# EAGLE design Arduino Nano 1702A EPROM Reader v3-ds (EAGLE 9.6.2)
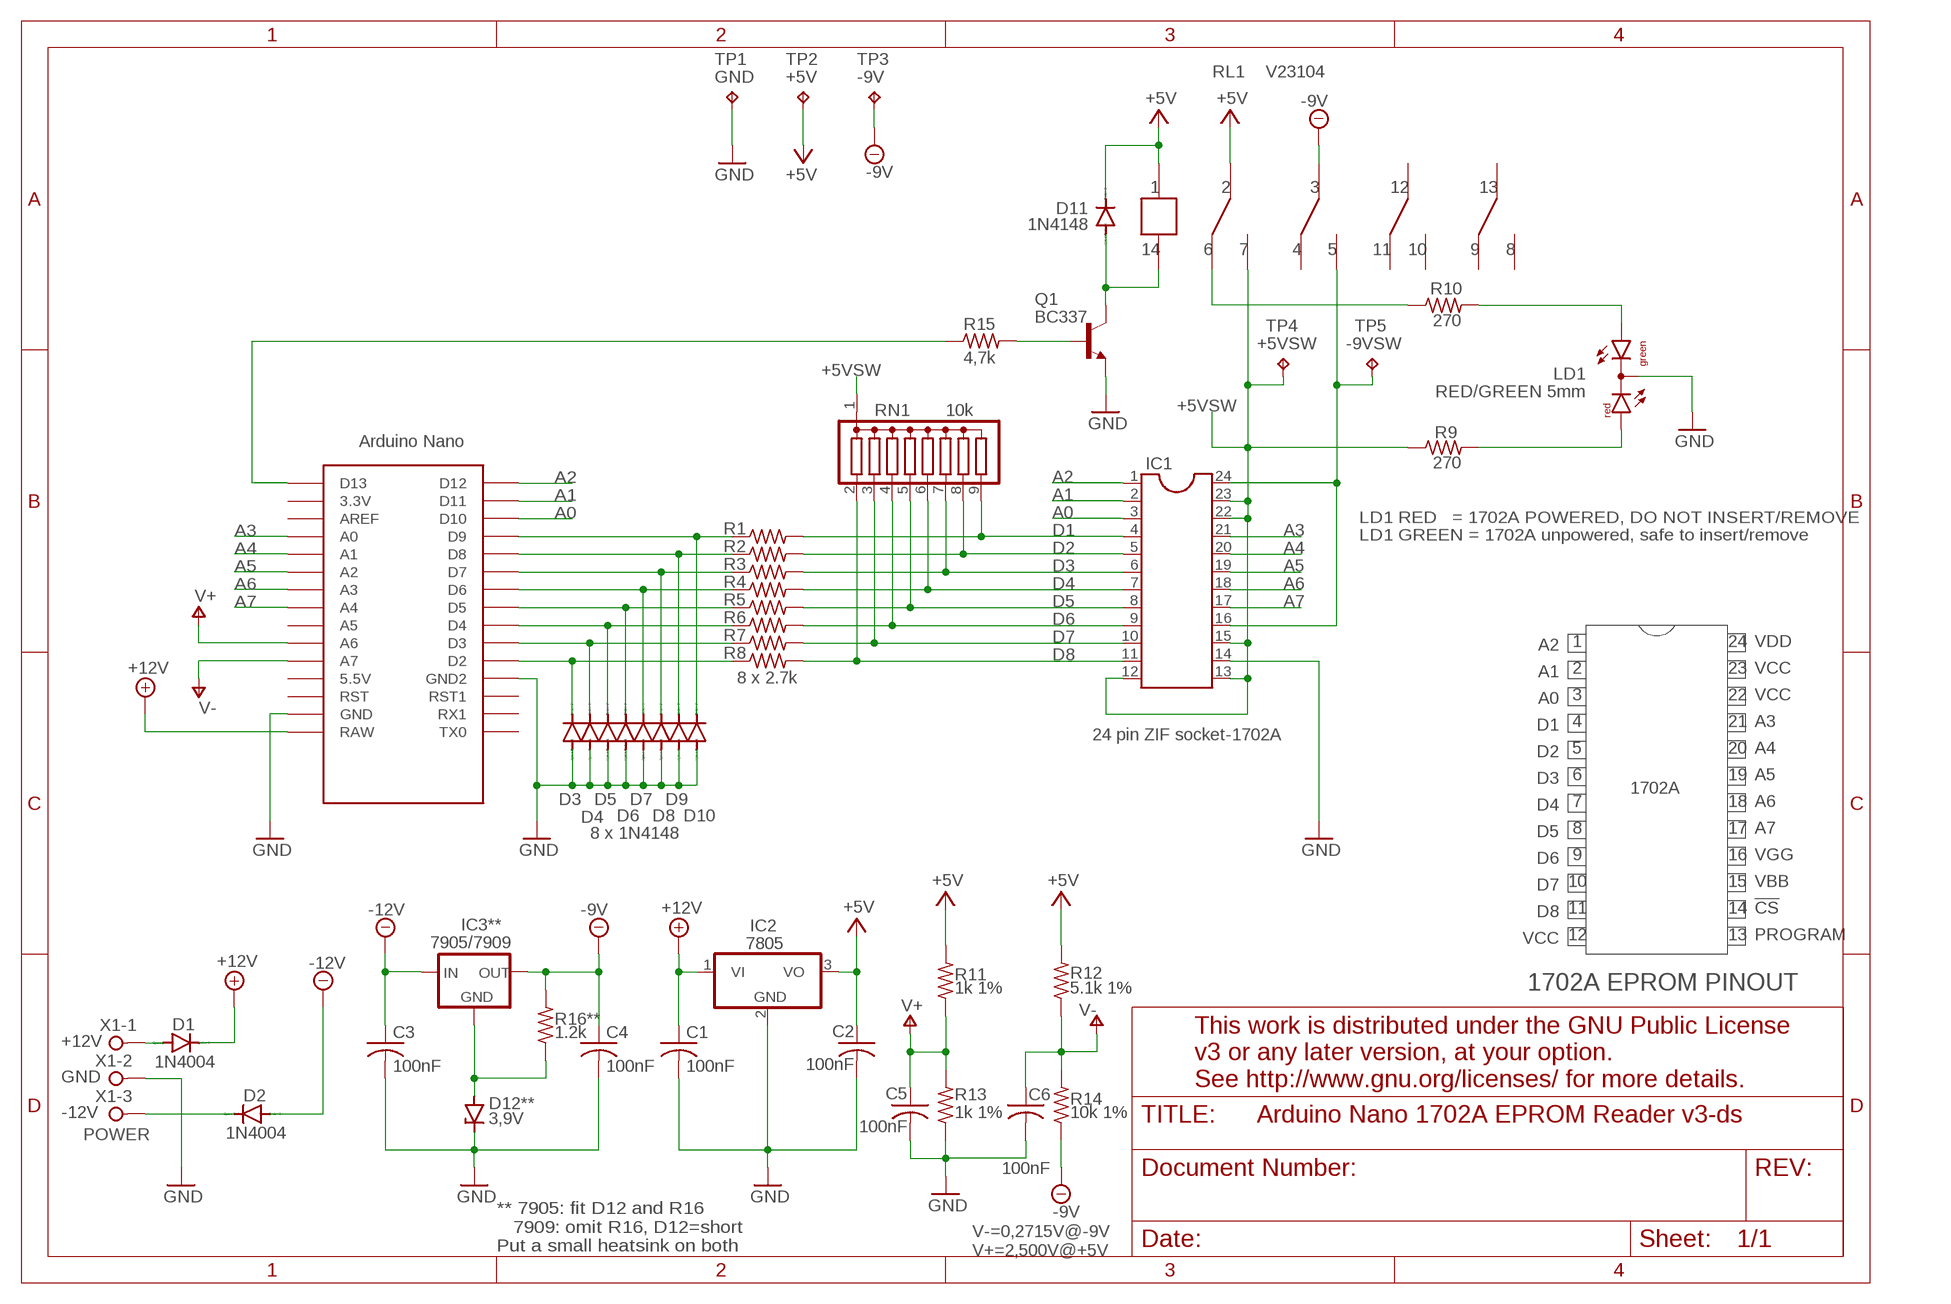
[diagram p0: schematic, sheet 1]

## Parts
C1  100nF  RCL_C-US050-025X075  [RCL_C050-025X075]
C2  100nF  RCL_C-US050-025X075  [RCL_C050-025X075]
C3  100nF  RCL_C-US050-025X075  [RCL_C050-025X075]
C4  100nF  RCL_C-US050-025X075  [RCL_C050-025X075]
C5  100nF  RCL_C-US050-025X075  [RCL_C050-025X075]
C6  100nF  RCL_C-US050-025X075  [RCL_C050-025X075]
D1  1N4004  ARDUINO-NANO-1702A-EPROM-READER-V2_1N4004  [ARDUINO-NANO-1702A-EPROM-READER-V2_DO41-10]
D2  1N4004  ARDUINO-NANO-1702A-EPROM-READER-V2_1N4004  [ARDUINO-NANO-1702A-EPROM-READER-V2_DO41-10]
D3  8 x 1N4148  DIODE_1N4148DO35-10  [DIODE_DO35-10]
D4  DIODE_1N4148DO35-10  [DIODE_DO35-10]
D5  DIODE_1N4148DO35-10  [DIODE_DO35-10]
D6  DIODE_1N4148DO35-10  [DIODE_DO35-10]
D7  DIODE_1N4148DO35-10  [DIODE_DO35-10]
D8  DIODE_1N4148DO35-10  [DIODE_DO35-10]
D9  DIODE_1N4148DO35-10  [DIODE_DO35-10]
D10  1N4148  DIODE_1N4148DO35-10  [DIODE_DO35-10]
D11  1N4148  DIODE_1N4148DO35-10  [DIODE_DO35-10]
D12**  3,9V  DIODE_ZPD  [DIODE_DO35Z10]
IC1  24 pin ZIF socket-1702A  IC-PACKAGE_DIL24-6  [IC-PACKAGE_DIL24-6]
IC2  7805  LINEAR_7805TV  [LINEAR_TO220V]
IC3**  7905/7909  V-REG_79XXS  [V-REG_79XXS]
LD1  RED/GREEN 5mm  LED_DUOLED-RG-C  [LED_DUOLED-C-5MM]
Q1  BC337  TRANSISTOR-NPN_BC237  [TRANSISTOR-NPN_TO92]
R1  RCL_R-US_0207/10  [RCL_0207/10]
R2  RCL_R-US_0207/10  [RCL_0207/10]
R3  RCL_R-US_0207/10  [RCL_0207/10]
R4  RCL_R-US_0207/10  [RCL_0207/10]
R5  RCL_R-US_0207/10  [RCL_0207/10]
R6  RCL_R-US_0207/10  [RCL_0207/10]
R7  RCL_R-US_0207/10  [RCL_0207/10]
R8  8 x 2.7k  RCL_R-US_0207/10  [RCL_0207/10]
R9  270  RCL_R-US_0207/10  [RCL_0207/10]
R10  270  RCL_R-US_0207/10  [RCL_0207/10]
R11  1k 1%  RCL_R-US_0207/10  [RCL_0207/10]
R12  5.1k 1%  RCL_R-US_0207/10  [RCL_0207/10]
R13  1k 1%  RCL_R-US_0207/10  [RCL_0207/10]
R14  10k 1%  RCL_R-US_0207/10  [RCL_0207/10]
R15  4,7k  RCL_R-US_0207/10  [RCL_0207/10]
R16**  1.2k  RCL_R-US_0207/10  [RCL_0207/10]
RL1  V23104  ARDUINO-NANO-1702A-EPROM-READER-V2_V23104  [ARDUINO-NANO-1702A-EPROM-READER-V2_V23104]
RN1  10k  G08R  [SIL9]
TP1  TPPAD1-13Y  [P1-13Y]
TP2  TPPAD1-13Y  [P1-13Y]
TP3  TPPAD1-13Y  [P1-13Y]
TP4  +5VSW  TPPAD1-13Y  [P1-13Y]
TP5  TPPAD1-13Y  [P1-13Y]
U$1  ARDUINO-CLONE_NANO  [ARDUINO-CLONE_NANO]
X1  POWER  CON-WAGO-508_W237-3E  [CON-WAGO-508_W237-3E]

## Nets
+5V: C2.1 D11.C IC2.3(VO) R11.2 R12.2 RL1.P$1 RL1.P$2 TP2.TP
+5VSW: IC1.12 IC1.13 IC1.15 IC1.22 IC1.23 R9.1 RL1.P$7 RN1.1 TP4.TP
+12V: C1.1 D1.C IC2.1(VI) U$1.RAW
-9V: C4.1 IC3**.OUT R14.1 R16**.2 RL1.P$3 TP3.TP
-9VSW: IC1.16 IC1.24 RL1.P$5 TP5.TP
-12V: C3.1 D2.A IC3**.IN
A0: IC1.3 U$1.D10
A1: IC1.2 U$1.D11
A2: IC1.1 U$1.D12
A3: IC1.21 U$1.A0
A4: IC1.20 U$1.A1
A5: IC1.19 U$1.A2
A6: IC1.18 U$1.A3
A7: IC1.17 U$1.A4
D1: IC1.4 R1.2 RN1.9
D2: IC1.5 R2.2 RN1.8
D3: IC1.6 R3.2 RN1.7
D4: IC1.7 R4.2 RN1.6
D5: IC1.8 R5.2 RN1.5
D6: IC1.9 R6.2 RN1.4
D7: IC1.10 R7.2 RN1.3
D8: IC1.11 R8.2 RN1.2
GND: C1.2 C2.2 C3.2 C4.2 C5.2 C6.2 D3.A D4.A D5.A D6.A D7.A D8.A D9.A D10.A D12**.C IC1.14 IC2.2(GND) LD1.C Q1.1(E) R13.1 TP1.TP U$1.GND U$1.GND1(GND2) X1.2
N$1: D1.A X1.1
N$2: D2.C X1.3
N$3: D12**.A IC3**.GND R16**.1
N$4: D11.A Q1.3(C) RL1.P$14
N$5: LD1.AR R9.2
N$6: D3.C R8.1 U$1.D2
N$7: D4.C R7.1 U$1.D3
N$8: D5.C R6.1 U$1.D4
N$9: D6.C R5.1 U$1.D5
N$10: D7.C R4.1 U$1.D6
N$11: D8.C R3.1 U$1.D7
N$12: D9.C R2.1 U$1.D8
N$13: D10.C R1.1 U$1.D9
N$15: LD1.AX(AG) R10.2
N$16: R10.1 RL1.P$6
N$17: Q1.2(B) R15.2
N$18: R15.1 U$1.D13
V+: C5.1 R11.1 R13.2 U$1.A6
V-: C6.1 R12.1 R14.2 U$1.A7
Unconnected: RL1.P$4 RL1.P$8 RL1.P$9 RL1.P$10 RL1.P$11 RL1.P$12 RL1.P$13 U$1.3.3V U$1.5V(5.5V) U$1.A5 U$1.AREF U$1.RST U$1.RST1 U$1.RX1 U$1.TX0

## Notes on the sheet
- LD1 RED   = 1702A POWERED, DO NOT INSERT/REMOVE
  LD1 GREEN = 1702A unpowered, safe to insert/remove
- A2
- 1 | 24 | VDD
- A1
- 2 | 23 | VCC
- A0
- 3 | 22 | VCC
- D1
- 4 | 21 | A3
- D2
- 5 | 20 | A4
- D3
- 6 | 19 | A5
- D4 | 1702A
- 7 | 18 | A6
- D5
- 8 | 17 | A7
- D6
- 9 | 16 | VGG
- D7
- 10 | 15 | VBB
- D8
- 11 | 14 | !CS!
- VCC
- 12 | 13 | PROGRAM
- 1702A EPROM PINOUT
- +12V
- GND
- This work is distributed under the GNU Public License
  v3 or any later version, at your option.
  See http://www.gnu.org/licenses/ for more details.
- -12V
- ** 7905: fit D12 and R16
     7909: omit R16, D12=short
  Put a small heatsink on both
- V-=0,2715V@-9V
  V+=2,500V@+5V

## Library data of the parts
C1-C6 = Arduino Nano 1702A EPROM Reader v3:RCL_C-US: CAPACITOR, American symbol; SPICEPREFIX: C
D1 D2 = Arduino Nano 1702A EPROM Reader v3:ARDUINO-NANO-1702A-EPROM-READER-V2_1N4004: DIODE
D3-D11 = Arduino Nano 1702A EPROM Reader v3:DIODE_1N4148: DIODE
D12** = Arduino Nano 1702A EPROM Reader v3:DIODE_ZPD: Z DIODE
IC1 = Arduino Nano 1702A EPROM Reader v3:IC-PACKAGE_DIL24: Dual In Line
IC2 = Arduino Nano 1702A EPROM Reader v3:LINEAR_78*: Positive VOLTAGE REGULATOR Source: http://cache.national.com/ds/LM/LM78L05.pdf http://www.fairchildsemi.com/ds/LM/LM7805.pdf
IC3** = Arduino Nano 1702A EPROM Reader v3:V-REG_79XXS: VOLTAGE REGULATOR
LD1 = Arduino Nano 1702A EPROM Reader v3:LED_DUOLED-RG-C: DUO LED 2 colors (red/green), 5 mm, round, common Cathode www.ligitek.com or other producers.
Q1 = Arduino Nano 1702A EPROM Reader v3:TRANSISTOR-NPN_BC237: NPN Transistor
R1-R15 R16** = Arduino Nano 1702A EPROM Reader v3:RCL_R-US_: RESISTOR, American symbol; SPICEPREFIX: R
RL1 = Arduino Nano 1702A EPROM Reader v3:ARDUINO-NANO-1702A-EPROM-READER-V2_V23104
RN1 = resistor-sil:G08R: SIL RESISTOR; OC_FARNELL: unknown; OC_NEWARK: unknown
TP1 = testpad:TP: Test pad; TP_SIGNAL_NAME: GND
TP2 = testpad:TP: Test pad; TP_SIGNAL_NAME: +5V
TP3 = testpad:TP: Test pad; TP_SIGNAL_NAME: -9V
TP4 = testpad:TP: Test pad; TP_SIGNAL_NAME: +5VSW
TP5 = testpad:TP: Test pad; TP_SIGNAL_NAME: -9VSW
U$1 = Arduino Nano 1702A EPROM Reader v3:ARDUINO-CLONE_NANO: Arduino Nano
X1 = Arduino Nano 1702A EPROM Reader v3:CON-WAGO-508_W237-3E: WAGO SREW CLAMP; OC_FARNELL: unknown; OC_NEWARK: unknown

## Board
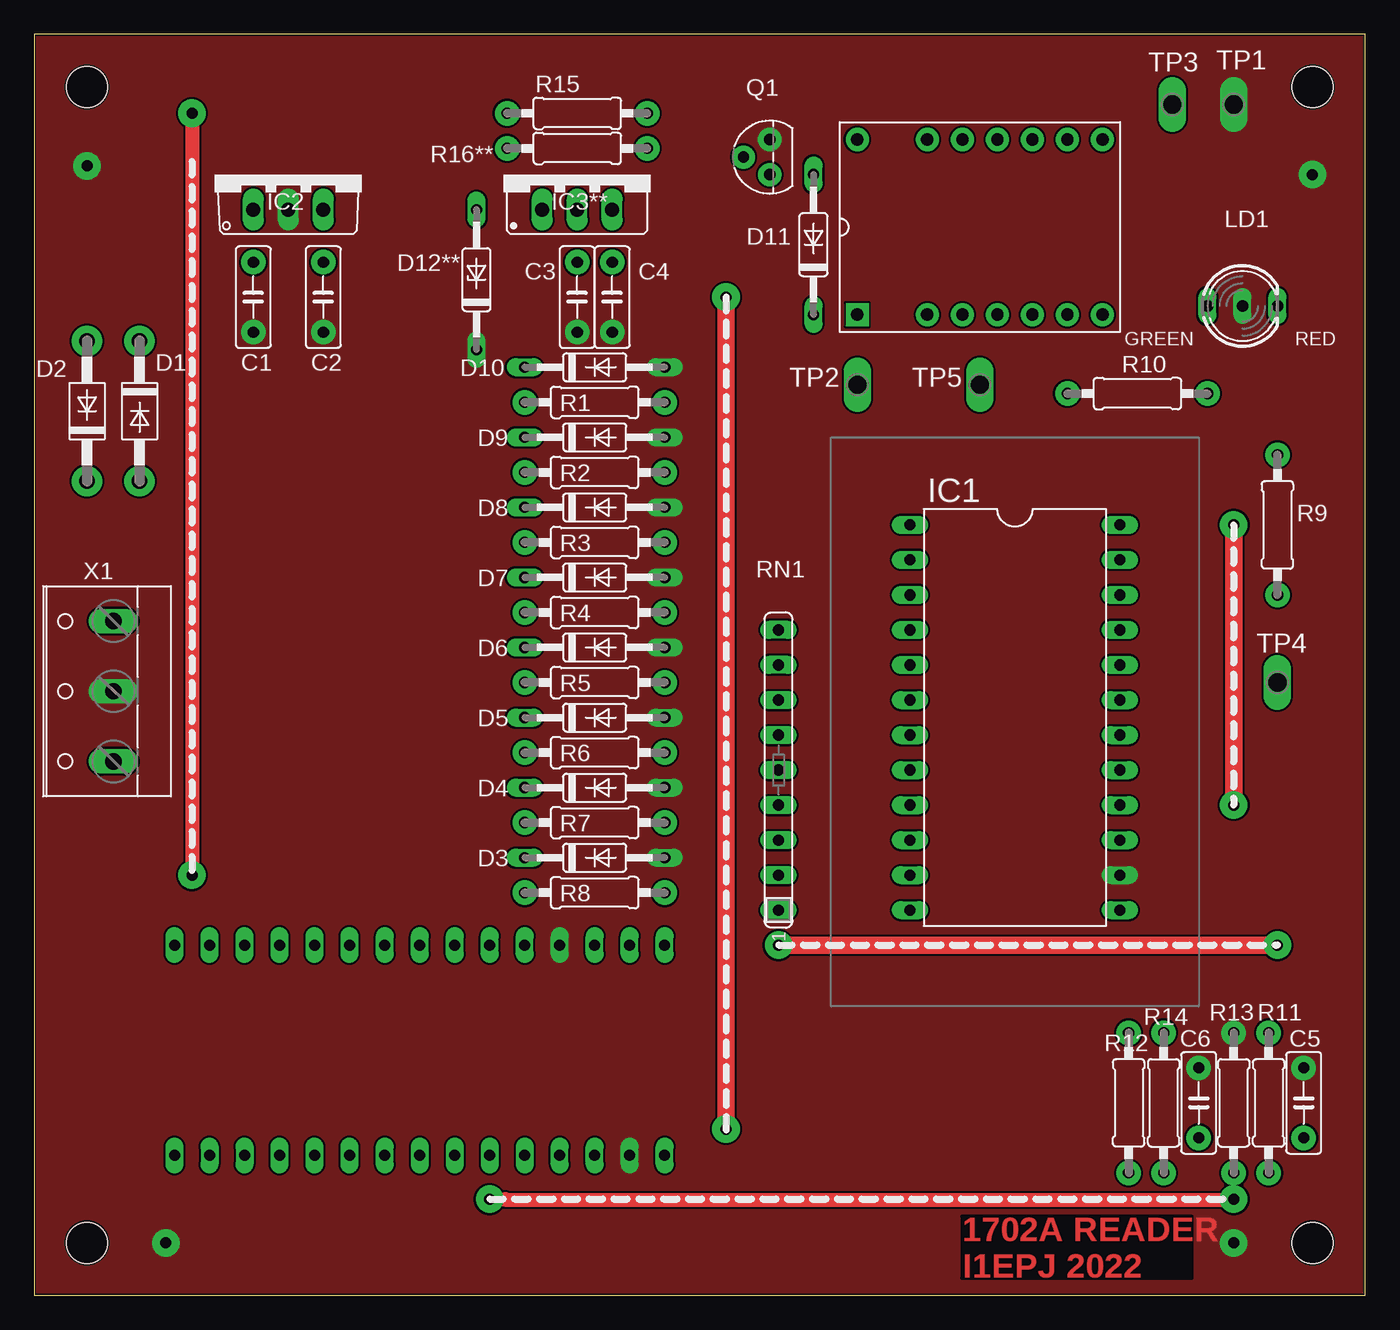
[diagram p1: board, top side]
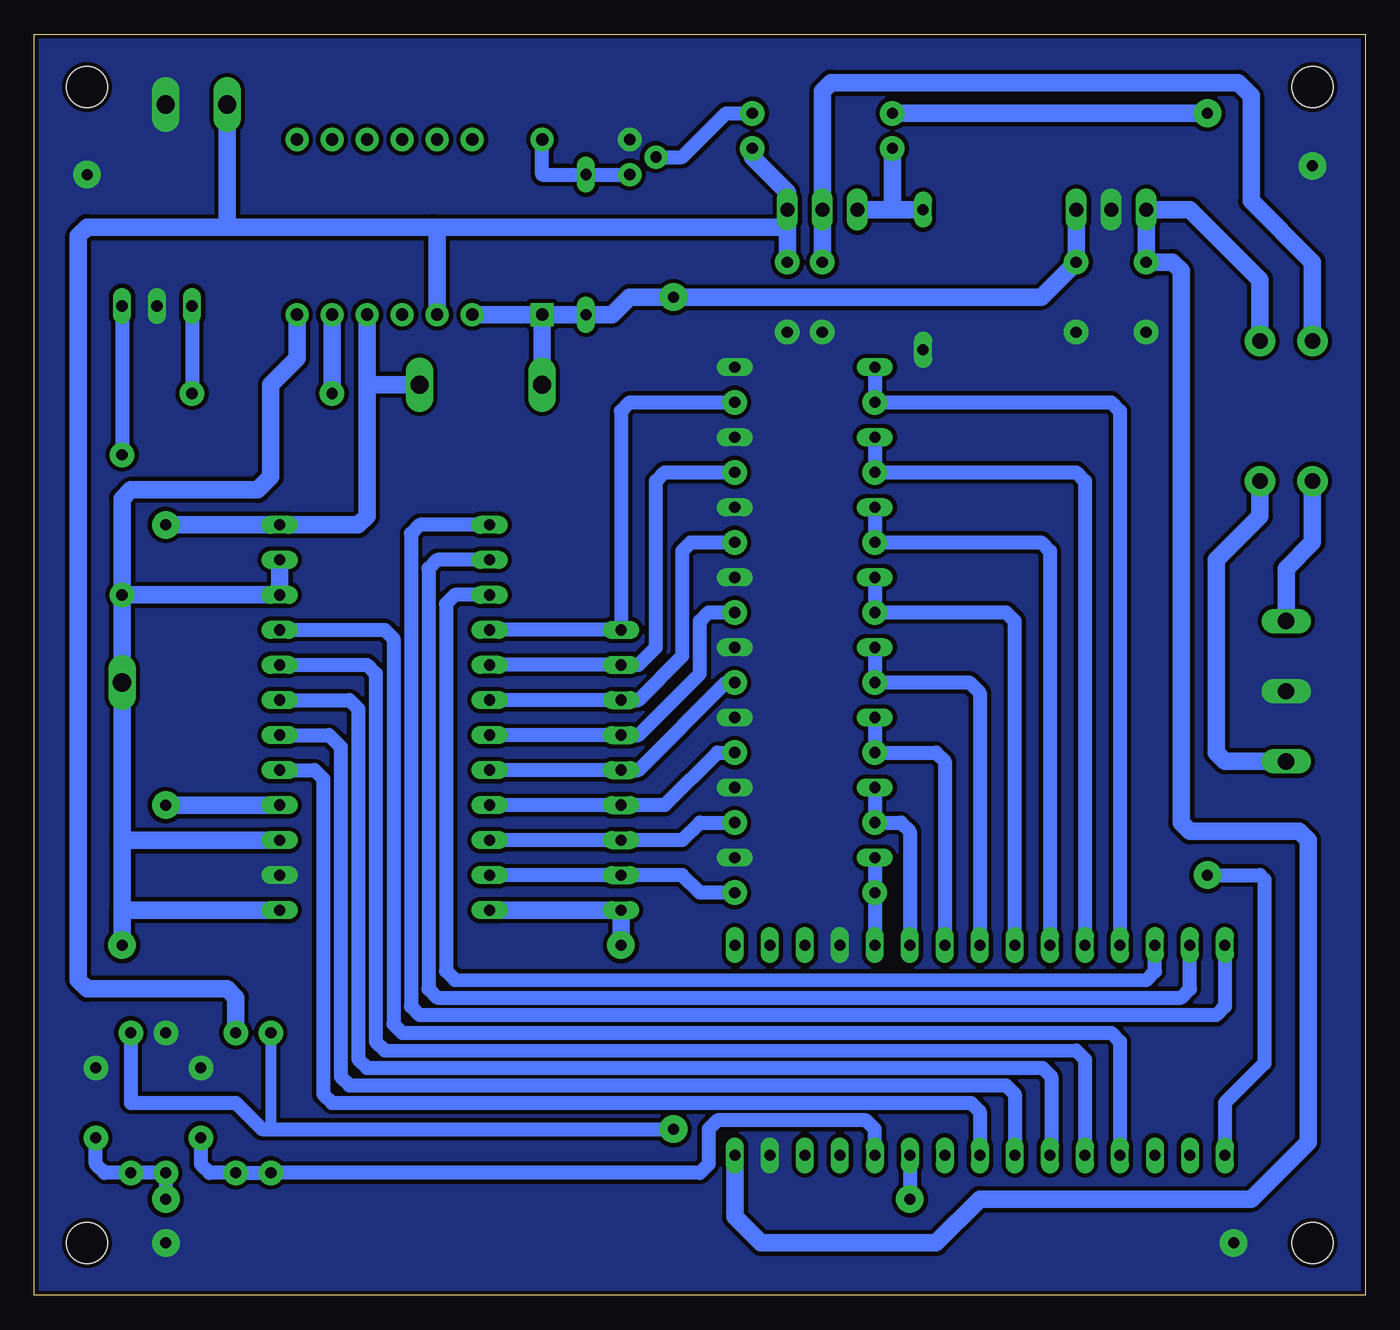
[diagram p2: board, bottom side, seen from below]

Size 96.52 x 91.44 mm. Coordinates in mm from the lower left corner, seen from the top.
Outline: 0,0 96.52,0 96.52,91.44 0,91.44 0,0
Copper layers (1*16): Top 0.035mm / dielectric 1.5mm / Bottom 0.035mm
Design rules "default *": minimum track width 6mil, minimum drill 0.35mm, track to track 6mil, track to pad 6mil, pad to pad 6mil, via to via 6mil, smd to smd 6mil, copper to edge 5mil, drill to drill 6mil, minimum pad ring 10mil, minimum via ring 8mil, stop-mask expansion 4mil, vias tented up to drill 0mil, thermal gap 0mil
Holes 3 mm at 92.71,3.81 3.81,3.81 3.81,87.63 92.71,87.63

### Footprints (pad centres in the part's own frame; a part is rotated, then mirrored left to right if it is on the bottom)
RCL_C050-025X075 = drill 0.813 pad 1.778: 1 -2.54,0; 2 2.54,0
ARDUINO-NANO-1702A-EPROM-READER-V2_DO41-10 = drill 1.118 pad 2.184: A 5.08,0; C -5.08,0
DIODE_DO35-10 = drill 0.813 long: A 5.08,0; C -5.08,0
DIODE_DO35Z10 = drill 0.813 long: A 5.08,0; C -5.08,0
IC-PACKAGE_DIL24-6 = drill 0.813 long: 1 -13.97,-7.62; 2 -11.43,-7.62; 3 -8.89,-7.62; 4 -6.35,-7.62; 5 -3.81,-7.62; 6 -1.27,-7.62; 7 1.27,-7.62; 8 3.81,-7.62; 9 6.35,-7.62; 10 8.89,-7.62; 11 11.43,-7.62; 12 13.97,-7.62; 13 13.97,7.62; 14 11.43,7.62; 15 8.89,7.62; 16 6.35,7.62; 17 3.81,7.62; 18 1.27,7.62; 19 -1.27,7.62; 20 -3.81,7.62; 21 -6.35,7.62; 22 -8.89,7.62; 23 -11.43,7.62; 24 -13.97,7.62
LINEAR_TO220V = drill 1.016 long: 1 -2.54,-2.54; 2 0,-2.54; 3 2.54,-2.54
V-REG_79XXS = drill 1.016 long: GND -2.54,-2.54; IN 0,-2.54; OUT 2.54,-2.54
LED_DUOLED-C-5MM = drill 0.813 long: AR 2.54,0; AX -2.54,0; C 0,0
TRANSISTOR-NPN_TO92 = drill 0.813 pad 1.676: 1 1.27,0; 2 0,1.905; 3 -1.27,0
RCL_0207/10 = drill 0.813 pad 1.778: 1 -5.08,0; 2 5.08,0
ARDUINO-NANO-1702A-EPROM-READER-V2_V23104 = drill 0.9 pad 1.676 square: P$1 -10.16,0 | drill 0.9 pad 1.676: P$2 -5.08,0; P$3 -2.54,0; P$4 0,0; P$5 2.54,0; P$6 5.08,0; P$7 7.62,0; P$8 7.62,12.7; P$9 5.08,12.7; P$10 2.54,12.7; P$11 0,12.7; P$12 -2.54,12.7; P$13 -5.08,12.7; P$14 -10.16,12.7
SIL9 = drill 0.813 long: 1 -10.16,0; 2 -7.62,0; 3 -5.08,0; 4 -2.54,0; 5 0,0; 6 2.54,0; 7 5.08,0; 8 7.62,0; 9 10.16,0
P1-13Y = drill 1.321 pad 1.905 long: TP 0,0
ARDUINO-CLONE_NANO = drill 0.8 long: 3.3V -10.16,24.13; 5V -10.16,-1.27; A0 -10.16,19.05; A1 -10.16,16.51; A2 -10.16,13.97; A3 -10.16,11.43; A4 -10.16,8.89; A5 -10.16,6.35; A6 -10.16,3.81; A7 -10.16,1.27; AREF -10.16,21.59; D2 5.08,1.27; D3 5.08,3.81; D4 5.08,6.35; D5 5.08,8.89; D6 5.08,11.43; D7 5.08,13.97; D8 5.08,16.51; D9 5.08,19.05; D10 5.08,21.59; D11 5.08,24.13; D12 5.08,26.67; D13 -10.16,26.67; GND -10.16,-6.35; GND1 5.08,-1.27; RAW -10.16,-8.89; RST -10.16,-3.81; RST1 5.08,-3.81; RX1 5.08,-6.35; TX0 5.08,-8.89
CON-WAGO-508_W237-3E = drill 1.194 long: 1 -5.08,-0.635; 2 0,-0.635; 3 5.08,-0.635

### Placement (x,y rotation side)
C1  15.88,72.39 270 top
C2  20.95,72.39 270 top
C3  39.37,72.39 270 top
C4  41.91,72.39 270 top
C5  92.08,13.97 90 top
C6  84.45,13.97 90 top
D1  7.62,64.14 270 top
D2  3.81,64.14 90 top
D3  40.64,31.75 0 top
D4  40.64,36.83 0 top
D5  40.64,41.91 0 top
D6  40.64,46.99 0 top
D7  40.64,52.07 0 top
D8  40.64,57.15 0 top
D9  40.64,62.23 0 top
D10  40.64,67.31 0 top
D11  56.52,76.2 90 top
D12**  32.07,73.66 90 top
IC1  71.12,41.91 270 top
IC2  18.41,81.28 0 top
IC3**  39.37,81.28 0 top
LD1  87.63,71.75 0 top
Q1  53.34,82.55 90 top
R1  40.64,64.77 0 top
R2  40.64,59.69 0 top
R3  40.64,54.61 0 top
R4  40.64,49.53 0 top
R5  40.64,44.45 0 top
R6  40.64,39.37 0 top
R7  40.64,34.29 0 top
R8  40.64,29.21 0 top
R9  90.17,55.88 90 top
R10  80.01,65.41 0 top
R11  89.53,13.97 90 top
R12  79.38,13.97 90 top
R13  87,13.97 270 top
R14  81.92,13.97 270 top
R15  39.37,85.72 0 top
R16**  39.37,83.19 0 top
RL1  69.85,71.12 0 top
RN1  53.98,38.1 90 top
TP1  87,86.36 0 top
TP2  59.69,66.04 0 top
TP3  82.55,86.36 0 top
TP4  90.17,44.45 180 top
TP5  68.58,66.04 0 top
U$1  36.83,20.32 90 top
X1  5.08,43.81 90 top

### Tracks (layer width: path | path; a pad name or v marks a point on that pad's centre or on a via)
+5V  (via drill 0.8 pad 2)
  Top 1.27: v50.16,72.39 v50.16,12.06
  Bottom 0.813: R12.2 79.38,12.06
  Bottom 1.016: R11.2 89.53,13.97 81.92,13.97 80.01,12.06 79.38,12.06 v50.16,12.06
  Bottom 1.27: IC2.3 C2.1 23.5,72.39 v50.16,72.39 53.34,72.39 54.61,71.12 D11.C RL1.P$1 | RL1.P$1 RL1.P$2 | TP2.TP RL1.P$1
+5VSW  (via drill 0.8 pad 2)
  Top 1.27: v90.17,25.4 v53.98,25.4
  Bottom 1.27: IC1.23 IC1.22 R9.1 | 90.17,33.02 90.17,27.94 | 90.17,33.02 IC1.15 | RL1.P$7 77.47,67.94 79.38,66.04 79.38,59.37 80.33,58.42 89.53,58.42 90.17,57.78 R9.1 | v53.98,25.4 RN1.1 IC1.12 | v90.17,25.4 90.17,27.94 | IC1.13 90.17,27.94 | R9.1 TP4.TP 90.17,33.02
+12V
  Bottom 1.27: U$1.RAW 45.72,5.71 43.81,3.81 31.11,3.81 27.94,6.99 8.26,6.99 4.13,11.11 4.13,33.02 4.76,33.66 12.7,33.66 13.34,34.29 13.34,74.3 13.97,74.93 C1.1 IC2.1 12.7,78.74 7.62,73.66 D1.C
-9V
  Bottom 1.27: 82.55,77.47 67.63,77.47 | 67.63,77.47 41.91,77.47 C4.1 IC3**.OUT 41.91,80.01 44.45,82.55 R16**.2 | 82.55,77.47 92.71,77.47 93.34,76.83 93.34,22.86 92.71,22.23 82.55,22.23 81.92,21.59 R14.1 | RL1.P$3 67.31,77.15 67.63,77.47 | TP3.TP 82.55,77.47
-9VSW  (via drill 0.8 pad 2)
  Top 1.27: v87,55.88 v87,35.56
  Bottom 1.27: 72.39,66.04 72.39,56.52 73.03,55.88 IC1.24 v87,55.88 | 72.39,66.04 RL1.P$5 | v87,35.56 IC1.16 | TP5.TP 72.39,66.04
-12V
  Bottom 1.27: C3.1 IC3**.IN 39.37,87.31 38.73,87.95 9.21,87.95 8.26,87 8.26,79.38 3.81,74.93 D2.A
A0
  Bottom 1.016: IC1.3 66.03,50.8 66.67,50.15 66.67,23.54 66.02,22.88 15.88,22.86 15.24,23.5 U$1.D10
A1
  Bottom 1.016: IC1.2 67.31,53.34 67.94,52.7 67.94,22.23 67.31,21.59 13.34,21.59 12.7,22.23 U$1.D11
A2
  Bottom 1.016: IC1.1 68.58,55.88 69.22,55.24 69.22,20.95 68.58,20.32 10.79,20.32 10.16,20.95 U$1.D12
A3
  Bottom 1.016: IC1.21 71.12,48.26 70.48,47.62 70.48,19.68 69.85,19.05 18.41,19.05 17.78,18.41 U$1.A0
A4
  Bottom 1.016: IC1.20 72.39,45.72 71.75,45.09 71.75,18.41 71.12,17.78 20.95,17.76 20.32,17.12 U$1.A1
A5
  Bottom 1.016: IC1.19 73.66,43.18 73.03,42.55 73.03,17.14 72.39,16.51 23.39,16.51 22.76,15.88 22.76,10.26 U$1.A2
A6
  Bottom 1.016: U$1.A3 25.4,14.61 26.04,15.24 73.66,15.24 74.3,15.88 74.3,39.78 75.16,40.64 IC1.18
A7
  Bottom 1.016: IC1.17 76.2,38.1 75.56,37.47 75.56,14.61 74.93,13.97 28.57,13.97 27.94,13.34 U$1.A4
D1
  Bottom 1.016: R1.2 53.34,64.77 53.98,64.14 RN1.9 IC1.4
D2
  Bottom 1.016: R2.2 50.8,59.69 51.44,59.05 51.44,46.99 52.7,45.72 RN1.8 IC1.5
D3
  Bottom 1.016: R3.2 48.9,54.61 49.53,53.98 49.53,46.35 52.7,43.18 RN1.7 IC1.6
D4
  Bottom 1.016: R4.2 47.62,49.53 48.26,48.9 48.26,45.09 52.7,40.64 RN1.6 IC1.7
D5
  Bottom 1.016: R5.2 46.35,44.45 52.7,38.1 RN1.5 IC1.8
D6
  Bottom 1.016: R6.2 46.99,39.37 50.8,35.56 RN1.4 IC1.9
D7
  Bottom 1.016: R7.2 48.26,34.29 49.53,33.02 RN1.3 IC1.10
D8
  Bottom 1.016: R8.2 48.26,29.21 49.53,30.48 RN1.2 IC1.11
GND  (via drill 0.8 pad 2)
  other vias: 3.81,81.92 92.71,81.28 9.53,3.81 87,3.81
  pour Bottom (isolate 0.305): 0,91.44 0,0 96.52,0 96.52,91.44
  pour Top: 0,91.44 0,0 96.52,0 96.52,91.44
N$1
  Bottom 1.27: X1.1 10.16,38.73 10.79,39.37 10.79,53.34 7.62,56.52 D1.A
N$2
  Bottom 1.27: D2.C 3.81,54.61 5.71,52.7 X1.3
N$3
  Bottom 1.27: D12**.A 34.29,78.74 | 34.29,78.74 IC3**.GND | R16**.1 34.29,78.74
N$4
  Bottom 1.016: Q1.3 D11.A 59.69,81.28 RL1.P$14
N$5
  Bottom 1.016: LD1.AR R9.2
N$6
  Bottom 1.016: R8.1 D3.C U$1.D2
N$7
  Bottom 1.016: D4.C R7.1 33.66,34.29 33.02,33.66 U$1.D3
N$8
  Bottom 1.016: D5.C R6.1 31.11,39.37 30.48,38.73 U$1.D4
N$9
  Bottom 1.016: D6.C R5.1 28.7,44.45 27.94,43.69 U$1.D5
N$10
  Bottom 1.016: D7.C R4.1 26.04,49.53 25.4,48.9 U$1.D6
N$11
  Bottom 1.016: D8.C R3.1 23.5,54.61 22.86,53.98 U$1.D7
N$12
  Bottom 1.016: D9.C R2.1 20.95,59.69 20.32,59.05 U$1.D8
N$13
  Bottom 1.016: D10.C R1.1 18.41,64.77 17.78,64.14 U$1.D9
N$15
  Bottom 1.016: LD1.AX R10.2
N$16
  Bottom 1.27: R10.1 RL1.P$6
N$17
  Bottom 1.016: R15.2 46.35,85.72 49.53,82.55 Q1.2
N$18  (via drill 0.8 pad 2)
  Top 1.016: v11.43,85.72 v11.43,30.48
  Bottom 1.016: v11.43,30.48 7.62,30.48 7.3,30.16 7.3,16.83 10.16,13.97 U$1.D13
  Bottom 1.27: R15.1 v11.43,85.72
V+  (via drill 0.8 pad 2)
  Top 1.016: v87,6.99 87.06,6.92 34.23,6.92 34.16,6.99 v33.02,6.99
  Bottom 1.016: U$1.A6 v33.02,6.99 | v87,6.99 R13.2 R11.1 91.44,8.89 92.08,9.53 C5.1
V-
  Bottom 1.016: U$1.A7 35.56,12.06 36.2,12.7 46.99,12.7 47.62,12.06 47.62,9.53 48.26,8.89 R12.1 R14.2 83.82,8.89 84.45,9.53 C6.1

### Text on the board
Top: 1702A READER / I1EPJ 2022
tPlace: GREEN | RED
tDocu: -12V | GND | +12V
